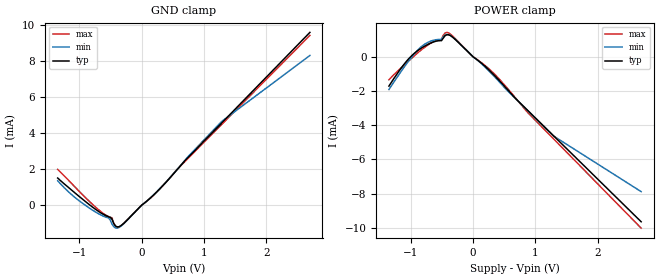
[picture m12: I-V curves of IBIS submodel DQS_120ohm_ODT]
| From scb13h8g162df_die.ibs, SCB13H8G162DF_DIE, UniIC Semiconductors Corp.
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|   Submodel DQS_120ohm_ODT
[Submodel] DQS_120ohm_ODT
Submodel_type Dynamic_clamp
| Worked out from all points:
|   GND clamp passes 1 mA (typ) near -0.28 V on its own axis
|   POWER clamp passes 1 mA (typ) near -0.28 V on its own axis
[GND_clamp]
|Voltage   I(typ)   I(min)   I(max)
-1.35V    1.503mA    1.349mA    1.982mA
-1.013V   502.6uA    259.6uA    794.1uA
-703mV    -327.9uA   -462.9uA   -228.6uA
-534mV    -650uA     -711.2uA   -638.8uA
-478mV    -786.6uA   -1.054mA   -707.6uA
-450mV    -1.019mA   -1.2mA     -1.001mA
-422mV    -1.158mA   -1.271mA   -1.17mA
-366mV    -1.204mA   -1.246mA   -1.214mA
253mV     772.7uA    781.1uA    763.6uA
562mV     1.944mA    1.956mA    1.963mA
1.294V    4.596mA    4.672mA    4.516mA
2.7V      9.593mA    8.31mA     9.425mA
[POWER_clamp]
|Voltage   I(typ)   I(min)   I(max)
-1.35V    -1.715mA   -1.914mA   -1.346mA
-1.069V   -268.4uA   -420.6uA   -361.9uA
-844mV    469.3uA    542.5uA    358.8uA
-675mV    806.4uA    918.3uA    798.9uA
-506mV    940.6uA    1.013mA    1.014mA
-450mV    1.221mA    1.272mA    1.385mA
-366mV    1.243mA    1.245mA    1.329mA
100nV     -188.8nA   -184.5nA   -196.7nA
338mV     -1.068mA   -1.135mA   -985.8uA
872mV     -3.113mA   -3.126mA   -3.234mA
1.294V    -4.62mA    -4.628mA   -4.798mA
2.7V      -9.64mA    -7.881mA   -10.01mA
